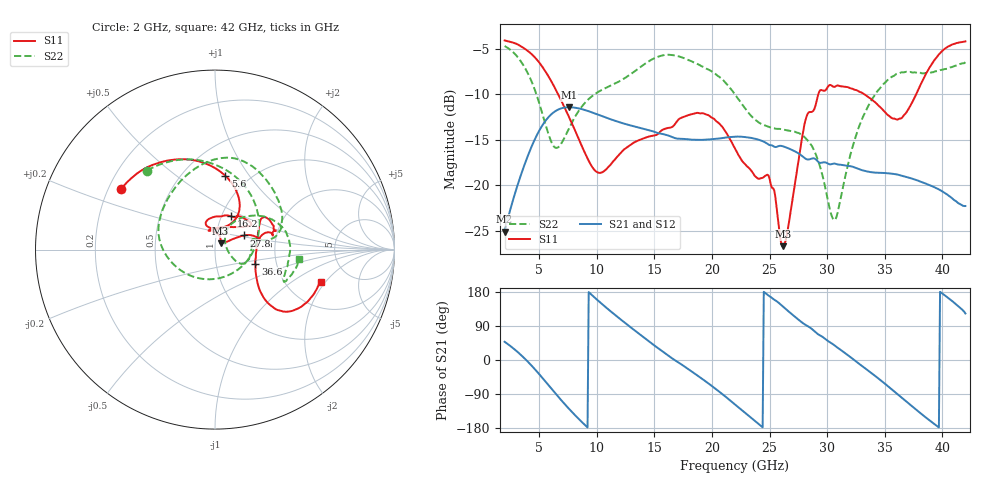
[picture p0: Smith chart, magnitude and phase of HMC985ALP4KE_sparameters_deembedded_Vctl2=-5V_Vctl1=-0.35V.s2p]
!s2p File: Measurements: S11, S21, S12, S22
# GHz S dB R 50.0
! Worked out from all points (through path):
!   401 points, 2 GHz to 42 GHz, reference 50 ohm
!   highest |S21| = -11.44 dB at 7.6 GHz (marker M1); lowest = -25.1 dB at 2 GHz (marker M2)
!   lowest |S11| = -26.7 dB at 26.2 GHz (marker M3), VSWR 1.10, Z = 53.1 + j3.65 ohm
!   |S11| at or under -10 dB: 6.637 GHz to 29.24 GHz (22.6 GHz wide, 126 % of centre); 33.2 GHz to 37.73 GHz (4.539 GHz wide, 12.8 % of centre)
!   |S22| runs from -23.8 to -4.7 dB; largest |S21 - S12| = 0.00027
!   S11 on the Smith chart (normalised r, x): 2 GHz: 0.25, +0.28; 5.6 GHz: 0.78, +0.78; 16.2 GHz: 1.11, +0.43; 27.8 GHz: 1.36, +0.22; 36.6 GHz: 1.55, -0.27; 42 GHz: 3.06, -1.80
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2  -4.11 147.2  -25.10 48.1  -25.11 48.1  -4.72 130.7
3.6  -4.89 120.5  -18.22 8.0  -18.22 8.0  -6.78 85.3
5.6  -7.63 82.1  -12.85 -58.7  -12.86 -58.7  -13.54 -4.3
6.5  -9.66 67.1  -11.80 -91.4  -11.81 -91.4  -15.91 -71.7
7.6  -12.54 56.8  -11.44 -129.2  -11.45 -129.2  -13.73 -138.0
8.7  -15.71 59.4  -11.65 -163.5  -11.66 -163.5  -11.38 -171.7
10.2  -18.65 87.8  -12.29 154.4  -12.30 154.4  -9.71 164.1
11.9  -16.71 109.9  -13.06 111.3  -13.07 111.3  -8.64 140.9
15.4  -14.27 76.7  -14.31 29.6  -14.32 29.6  -5.86 87.1
16.2  -13.71 64.0  -14.55 11.8  -14.55 11.8  -5.68 77.3
19.4  -12.20 34.6  -15.01 -55.2  -15.02 -55.2  -7.12 35.5
22  -15.97 52.2  -14.68 -117.3  -14.69 -117.3  -10.04 10.6
24.9  -18.93 102.4  -15.54 170.3  -15.54 170.4  -13.60 12.9
26.2  -26.71 48.0  -15.75 139.8  -15.76 139.9  -13.90 -1.8
27.8  -14.97 26.2  -16.77 99.4  -16.78 99.4  -14.48 -22.6
28.7  -11.94 12.3  -17.07 81.2  -17.07 81.2  -15.76 -28.8
30.7  -9.18 20.3  -17.65 37.0  -17.66 37.0  -23.80 23.5
32.9  -9.79 33.6  -18.31 -13.0  -18.31 -12.9  -13.14 51.6
35.4  -12.42 11.0  -18.72 -72.2  -18.72 -72.2  -8.33 21.6
36.6  -12.43 -19.7  -19.00 -102.6  -19.00 -102.6  -7.62 6.7
39.6  -5.81 -42.3  -20.40 -175.6  -20.41 -175.6  -7.48 -24.8
42  -4.21 -17.2  -22.30 122.7  -22.31 122.8  -6.50 -6.2
